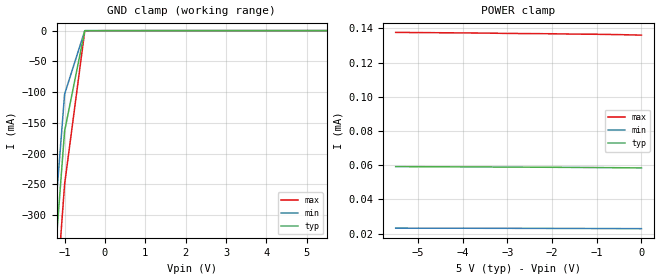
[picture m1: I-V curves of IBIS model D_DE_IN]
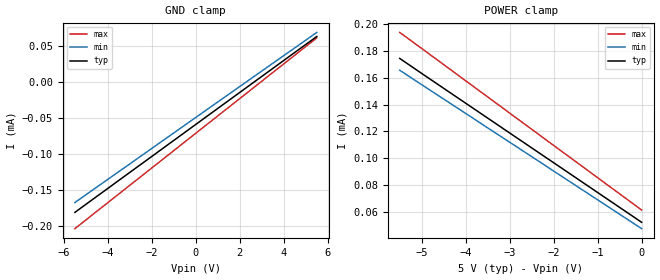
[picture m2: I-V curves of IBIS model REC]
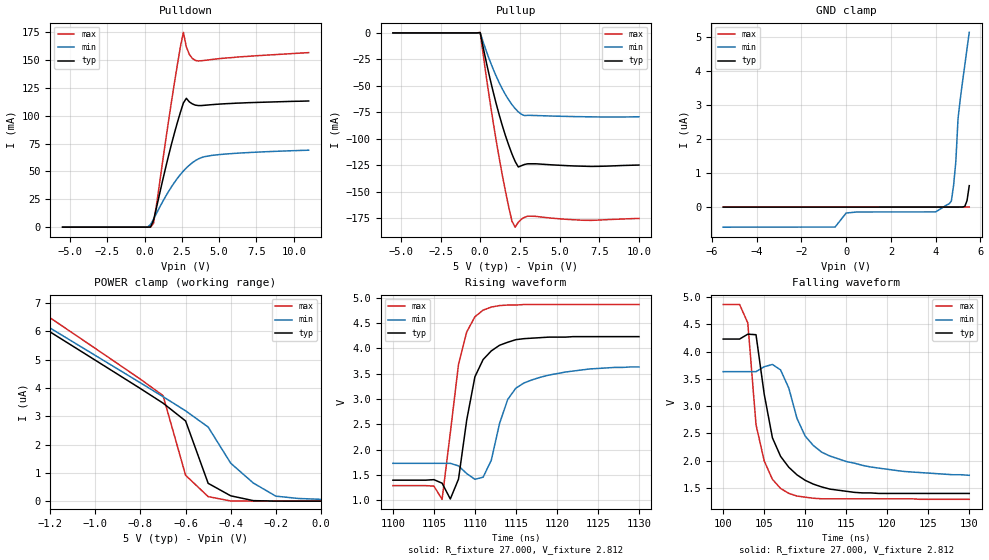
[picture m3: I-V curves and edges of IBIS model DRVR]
|   Texas Instruments Incorporated
|   Data Transmissions Products
|   IBIS Model for SN65HVD50
|   8D SOIC Package
[IBIS Ver]   3.2
[Comment char]   |_char
[File name]   hvd50.ibs
[File Rev]   1.0
[Date]   11Apr07
[Source]   File originated at Texas Instruments Incorporated.
   Data Transmission Products Group.
[Notes]
[Disclaimer]
(C) Copyright Texas Instruments Incorporated 2002
   All rights reserved
  Texas Instruments Incorporated hereby grants the user of this IBIS
model a non-exclusive, nontransferable license to use this IBIS model
under the following terms.  Before using this IBIS model, the user
should read this license.  If the user does not accept these terms,
the IBIS model should be returned to Texas Instruments within 30 days.
  The user is granted this license only to use the IBIS model and
is not granted rights to sell, load, rent, lease or license the IBIS
model in whole or in part, or in modified form to anyone other than
user.  User may modify the IBIS model to suit its specific applications
but rights to derivative works and such modifications shall belong to
Texas Instruments.
  This IBIS model is provided on an "AS IS" basis and Texas Instruments
makes absolutely no warranty with respect to the information contained
herein.  TEXAS INSTRUMENTS DISCLAIMS AND CUSTOMER WAIVES ALL WARRANTIES,
EXPRESS OR IMPLIED, INCLUDING WARRANTIES OF MERCHANTABILITY OR FITNESS
FOR A PARTICULAR PURPOSE. The entire risk as to quality and performance
is with the Customer. ACCORDINGLY, IN NO EVENT SHALL THE COMPANY BE LIABLE
FOR ANY DAMAGES, WHETHER IN CONTRACT OR TORT,INCLUDING ANY LOST PROFITS
OR OTHER INCIDENTAL, CONSEQUENTIAL, EXEMPLARY, OR PUNITIVE DAMAGES ARISING
OUT OF THE USE OR APPLICATION OF THE IBIS model provided in this package.
Further, Texas Instruments reserves the right to discontinue or make changes
without notice to any product herein to improve reliability, function, or
design. Texas Instruments does not convey any license under patent rights
or any other intellectual property rights, including those of third parties.
Contact Texas Instruments at ATTN:DATA TRANSMISSIONS
[Copyright]   Copyright 2002, Texas Instruments, All Rights Reserved
[Component]   HVD50D
[Manufacturer]  Texas Instruments Incorporated
[Package]
|   typ   min   max
R_pkg   0.071   0.050   0.091
L_pkg   2.203nH   1.540nH   2.930nH
C_pkg   0.465pF   0.385pF   0.609pF
[Pin]   signal_name   model_name   R_pin   L_pin   C_pin
1   VCC   POWER   0.091   2.615n   0.500p
2   R   RECEIVER_OUT   0.076   2.346n   0.483p
3   D   D_DE_IN   0.062   1.755n   0.395p
4   GND   GND   0.090   2.593n   0.498p
5   Y   DRVR   0.073   2.300n   0.480p
6   Z   DRVR   0.076   2.012n   0.407p
7   B   REC   0.050   1.540n   0.385p
8   A   REC   0.070   1.897n   0.412p
[Diff_pin]   inv_pin   vdiff   tdelay_typ   tdelay_min   tdelay_max
| The 'A' pin is Diff_pin and the 'B' pin is the inv_pin
5   6   0.200   0 0 0
7   8   0.200   0 0 0
| Models and submodels in the file (4): D_DE_IN (Input), REC (Input), DRVR (I/O), RECEIVER_OUT (3-state)
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|   Driver Input / Driver Enable / Model
[Model]   D_DE_IN
Model_type   Input
|Signals   D
Vinh = 2.0
Vinl = 0.8
|   typ   min   max
C_comp   23pF   19pF   27pF
|   typ   min   max
[Temperature Range]   27   -40   85
[Voltage range]   5.0V   4.5V   5.5V
[GND_clamp]
|   Voltage   I(typ)   I(min)   I(max)
-5.5V     -3.894A    -3.744A    -4.095A
-1.5V     -596.3mA   -523.6mA   -696.4mA
-1V       -163.5mA   -103.3mA   -250mA
-500mV    -18.38uA   -37.25uA   -400.5uA
5.5V      58.51uA    136uA      22.98uA
[Power_clamp]
| Note that the[POWER_clamp]voltage table is referenced to Vcc
| and is calculated using Vtable=Vcc - Vmeasured.
|   Voltage   I(typ)   I(min)   I(max)
-5.5V     59.15uA    23.21uA    137.6uA
-5V       59.11uA    23.19uA    137.5uA
-4.5V     59.06uA    23.17uA    137.4uA
-4V       59.01uA    23.15uA    137.3uA
-3.5V     58.95uA    23.12uA    137.2uA
-3V       58.9uA     23.1uA     137uA
-2.5V     58.83uA    23.07uA    136.9uA
-2V       58.77uA    23.04uA    136.8uA
-1.5V     58.69uA    23.01uA    136.6uA
-1V       58.61uA    22.98uA    136.5uA
-500mV    58.51uA    22.94uA    136.3uA
0V        58.4uA     22.9uA     136uA
|   Receiver Input / Model
[Model]   REC
Model_type   Input
|Signals   A,B
Vinh = 2.0
Vinl = 0.8
|   typ   min   max
C_comp   3pF   2.5pF   3.5pF
|   typ   min   max
[Temperature Range]   27   -40   85
[Voltage range]   5.0V   4.5V   5.5V
[GND_clamp]
|   Voltage   I(typ)   I(min)   I(max)
-5.5V     -181.4uA   -167.7uA   -204uA
-3.5V     -136.8uA   -124.6uA   -155.7uA
1V        -36.71uA   -27.75uA   -47.12uA
5.5V      63.31uA    68.95uA    61.36uA
[Power_clamp]
| Note that the[POWER_clamp]voltage table is referenced to Vcc
| and is calculated using Vtable=Vcc - Vmeasured.
|   Voltage   I(typ)   I(min)   I(max)
-5.5V     174.4uA    165.6uA    193.8uA
-5V       163.2uA    154.8uA    181.8uA
-4.5V     152.1uA    144.1uA    169.8uA
-4V       141uA      133.4uA    157.7uA
-3.5V     129.9uA    122.6uA    145.7uA
-3V       118.8uA    111.9uA    133.6uA
-2.5V     107.7uA    101.2uA    121.6uA
-2V       96.62uA    90.42uA    109.5uA
-1.5V     85.52uA    79.68uA    97.5uA
-1V       74.41uA    68.95uA    85.45uA
-500mV    63.31uA    58.21uA    73.4uA
0V        52.2uA     47.47uA    61.36uA
|   Driver Output / Receiver Input Model
[Model]   DRVR
Model_type   I/O
| Signals   Y,Z
Vinl = 0.9V
Vinh = 2.8V
Vmeas = 1.7V   |Reference voltage for timing measurements
Cref = 50pF   |Timing specification test load capacitance value
Rref = 54   |Note: 54 Ohm load; single-ended configuration
|   Timing specification test load voltage
| variable   typ   min   max
C_comp   28pF   24pF   32pF
|   typ   min   max
[Temperature Range]   25.0   -40   85
[Voltage range]   5.0V   4.5V   5.5V
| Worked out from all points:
|   slope of the pulldown table from 0 to 0.75 V, typ, clamps not added: 50.7 ohm
|   slope of the pullup table from 0 to 0.75 V, typ, clamps not added: 14.5 ohm
|   rising waveform, R_fixture 27.000, V_fixture 2.812: 20-80 % time 2.2ns typ, 2.92ns min, 1.98ns max; typ from 1.4 V to 4.23 V
|   falling waveform, R_fixture 27.000, V_fixture 2.812: 20-80 % time 2.98ns typ, 4.49ns min, 1.78ns max; typ from 4.23 V to 1.4 V
[Pulldown]
|   Voltage   I(typ)   I(min)   I(max)
-5.5V     -10.66pA   -1.61nA    -2.66pA
200mV     102.2nA    81.88uA    446.1pA
400mV     121.7uA    2.397mA    2.576uA
600mV     6.248mA    7.209mA    3.471mA
1.8V      74.35mA    36.14mA    112.4mA
2.4V      103mA      47.21mA    161.8mA
2.6V      111.4mA    50.31mA    174.8mA
2.8V      115.6mA    53.11mA    161.7mA
3V        112.4mA    55.6mA     155mA
3.6V      109.1mA    61.2mA     149.1mA
5.5V      110.8mA    65.68mA    151.8mA
11V       113.2mA    69.05mA    156.6mA
[Pullup]
|   Voltage   I(typ)   I(min)   I(max)
| Note that the[Pullup]voltage table is referenced to Vcc
| and is calculated using Vtable=Vcc - Vmeasured.
-5.5V     2.4uA      2.144uA    2.981uA
0V        269.5uA    177uA      535.4uA
600mV     -42.03mA   -26mA      -63.31mA
1.2V      -77.48mA   -47.12mA   -118.3mA
1.6V      -97.35mA   -58.48mA   -150.1mA
2V        -114.2mA   -67.65mA   -177.6mA
2.2V      -121.3mA   -71.41mA   -183.3mA
2.4V      -126.5mA   -74.49mA   -178.7mA
2.8V      -124.1mA   -78.04mA   -173.9mA
3V        -123.5mA   -77.81mA   -172.9mA
6.5V      -125.8mA   -79.1mA    -176.8mA
10V       -124.7mA   -79.14mA   -175.1mA
[GND_clamp]
|   Voltage  I(typ)   I(min)   I(max)
| Outputs in High Impedance (off)
-5.5V     -1.17nA    -592nA     -1.094nA
-500mV    -651.3pA   -589.2nA   -574.5pA
0V        -526.7pA   -174.9nA   -522.6pA
4V        256.2pA    -142.8nA   173.6pA
4.6V      361.5pA    94.35nA    277.1pA
4.7V      380.1pA    176.4nA    294pA
4.8V      394.4pA    641.3nA    311.8pA
4.9V      418.3pA    1.34uA     326.9pA
5V        446.8pA    2.618uA    343.7pA
5.3V      18.21nA    4.177uA    389pA
5.4V      188.2nA    4.662uA    400.6pA
5.5V      629.7nA    5.145uA    417.4pA
[POWER_clamp]
|   Voltage  I(typ)   I(min)   I(max)
| Note that the [POWER_clamp] voltage table is referenced to Vcc
| and is calculated using Vtable = Vcc - Vmeasured.
| Outputs in Tri-state.
-5.5V     27.39uA    26.86uA    29.68uA
-1.5V     7.468uA    7.559uA    8.092uA
-1.4V     6.97uA     7.077uA    7.552uA
-1.3V     6.472uA    6.594uA    7.012uA
-800mV    3.975uA    4.177uA    4.305uA
-700mV    3.462uA    3.69uA     3.728uA
-600mV    2.832uA    3.19uA     913.7nA
-500mV    629.7nA    2.618uA    159.9nA
-400mV    188.2nA    1.34uA     5.888nA
-300mV    18.21nA    641.3nA    839.3pA
-200mV    1.35nA     176.4nA    418.3pA
0V        446.8pA    64.16nA    417.4pA
[Ramp]
|   typ   min   max
dV/dt_r   1.69V/2.2ns   1.12V/2.9ns   2.14V/2.0ns
dV/dt_f   1.70V/4.2ns   1.13V/4.7ns   2.16V/2.2ns
R_load = 27ohm | Note: The measurement is on a single-ended configuration
|   with 54ohm line-to-line.
[Rising Waveform]
R_fixture = 27.000
V_fixture = 2.812
V_fixture_min = 2.663
V_fixture_max = 3.070
C_fixture = 0.000
L_fixture = 0.000
|  time   V(typ)   V(min)   V(max)
1.1us     1.395V     1.728V     1.287V
1.105us   1.405V     1.728V     1.277V
1.106us   1.335V     1.728V     1.016V
1.107us   1.023V     1.728V     2.33V
1.108us   1.415V     1.677V     3.683V
1.11us    3.438V     1.412V     4.625V
1.111us   3.779V     1.453V     4.756V
1.114us   4.121V     2.991V     4.856V
1.115us   4.172V     3.215V     4.856V
1.13us    4.232V     3.633V     4.867V
[Falling Waveform]
R_fixture = 27.000
V_fixture = 2.812
V_fixture_min = 2.663
V_fixture_max = 3.070
C_fixture = 0.000
L_fixture = 0.000
|  time   V(typ)   V(min)   V(max)
100ns     4.232V     3.633V     4.867V
102ns     4.232V     3.633V     4.867V
103ns     4.322V     3.633V     4.528V
104ns     4.312V     3.633V     2.659V
105ns     3.22V      3.724V     1.993V
106ns     2.418V     3.765V     1.655V
107ns     2.076V     3.664V     1.486V
110ns     1.636V     2.448V     1.327V
112ns     1.515V     2.154V     1.297V
130ns     1.395V     1.728V     1.287V
